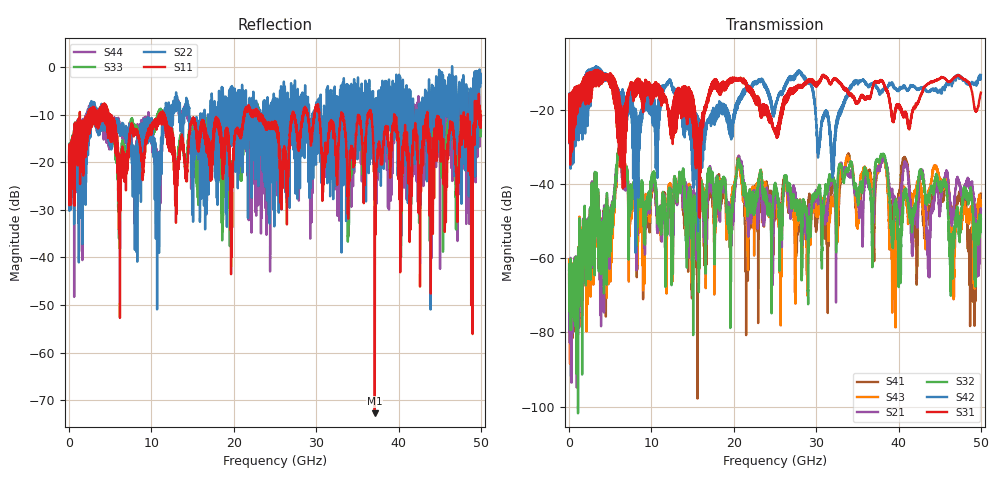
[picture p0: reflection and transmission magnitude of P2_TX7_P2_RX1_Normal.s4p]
!Keysight Technologies,N5225B,MY57041031,A.13.20.10
!Date: Friday, May 31, 2019 11:27:57
!Correction: S11(Full 4 Port(1,2,3,4))
!S12(Full 4 Port(1,2,3,4))
!S13(Full 4 Port(1,2,3,4))
!S14(Full 4 Port(1,2,3,4))
!S21(Full 4 Port(1,2,3,4))
!S22(Full 4 Port(1,2,3,4))
!S23(Full 4 Port(1,2,3,4))
!S24(Full 4 Port(1,2,3,4))
!S31(Full 4 Port(1,2,3,4))
!S32(Full 4 Port(1,2,3,4))
!S33(Full 4 Port(1,2,3,4))
!S34(Full 4 Port(1,2,3,4))
!S41(Full 4 Port(1,2,3,4))
!S42(Full 4 Port(1,2,3,4))
!S43(Full 4 Port(1,2,3,4))
!S44(Full 4 Port(1,2,3,4))
!S4P File: Measurements: <S11,S12,S13,S14>,
!<S21,S22,S23,S24>,
!<S31,S32,S33,S34>,
!<S41,S42,S43,S44>:
# Hz S  dB  R 50.0
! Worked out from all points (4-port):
!   5000 points, 10 MHz to 50 GHz, reference 50 ohm
!   strongest paths, dB at 10 MHz, 12.51 GHz, 25.01 GHz, 37.51 GHz, 50 GHz:
!     S31: -19.6, -21.0, -25.9, -12.8, -15.4
!     S42: -19.4, -14.2, -20.1, -14.4, -10.7
!     S32: -63.1, -52.0, -40.5, -33.5, -49.6
!     S21: -63.5, -49.0, -45.0, -35.7, -46.8
!     S43: -60.3, -55.4, -42.1, -37.2, -45.8
!     S41: -64.4, -53.0, -48.0, -36.8, -42.6
!   lowest |S11| = -72.7 dB at 37.12 GHz (marker M1), VSWR 1.00, Z = 50 + j0.0131 ohm
!   |S11| at or under -10 dB: 4.96 GHz to 10.98 GHz (6.02 GHz wide, 75.5 % of centre); 11.57 GHz to 21.26 GHz (9.683 GHz wide, 59 % of centre); 43.5 GHz to 47.91 GHz (4.406 GHz wide, 9.64 % of centre)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
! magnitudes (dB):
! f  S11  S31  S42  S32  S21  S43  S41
! 10 MHz  -20.1  -19.6  -19.4  -63.1  -63.5  -60.3  -64.4
! 6.14 GHz  -30.0  -18.0  -16.9  -30.1  -30.8  -30.2  -30.9
! 8.98 GHz  -22.6  -14.4  -20.4  -42.4  -43.7  -58.1  -56.1
! 37.12 GHz  -72.7  -12.6  -13.4  -36.5  -41.7  -40.6  -45.9
! 44.78 GHz  -13.9  -11.8  -15.4  -39.7  -42.7  -36.9  -37.7
! 49.17 GHz  -11.9  -18.8  -13.1  -57.3  -44.7  -65.6  -65.6
! 50 GHz  -11.1  -15.4  -10.7  -49.6  -46.8  -45.8  -42.6
